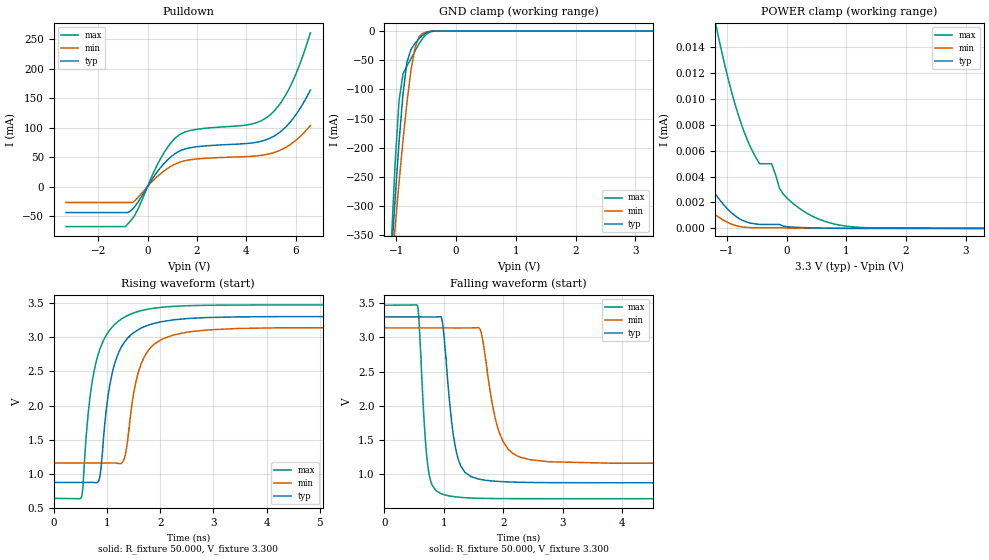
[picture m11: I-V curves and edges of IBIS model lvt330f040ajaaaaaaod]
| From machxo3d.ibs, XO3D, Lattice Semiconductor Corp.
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|   Model lvt330f040ajaaaaaaod
[Model] lvt330f040ajaaaaaaod
Model_type I/O_open_drain
Polarity   Non-Inverting
Enable   Active-Low
Vinl =  0.800V
Vinh =  2.000V
Vmeas =  1.650V
Cref =  0.0F
Rref = 10.00k
Vref = 3.30V
C_comp   4.200pF   3.800pF   7.500pF
[Temperature Range]   25.000   0.105k   -40.000
[Voltage Range]   3.300V   3.140V   3.470V
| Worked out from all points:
|   slope of the pulldown table from 0 to 0.495 V, typ, clamps not added: 16.2 ohm
|   GND clamp passes 1 mA (typ) near -0.43 V on its own axis
|   rising waveform, R_fixture 50.000, V_fixture 3.300: 20-80 % time 324ps typ, 329ps min, 328ps max; typ from 0.878 V to 3.3 V
|   falling waveform, R_fixture 50.000, V_fixture 3.300: 20-80 % time 180ps typ, 267ps min, 117ps max; typ from 3.3 V to 0.878 V
[Pulldown]
|Voltage   I(typ)   I(min)   I(max)
-3.3V     -43.98mA   -26.85mA   -67.81mA
-900mV    -43.98mA   -26.85mA   -67.81mA
-500mV    -33.06mA   -23.42mA   -47.39mA
600mV     35.86mA    24.47mA    52.84mA
1.2V      58.2mA     39.81mA    85.22mA
1.9V      67.18mA    46.53mA    96.69mA
4.2V      73.98mA    51.49mA    106.1mA
4.9V      81.14mA    55.32mA    119.6mA
5.4V      93.79mA    62.3mA     142.5mA
5.8V      110.5mA    71.89mA    171.7mA
6.2V      134mA      85.76mA    211.4mA
6.6V      164mA      103.9mA    261.1mA
[GND_clamp]
|Voltage   I(typ)   I(min)   I(max)
-3.3V     -4.507A    -3.482A    -6.263A
-1.089V   -398.4mA   -420.6mA   -374.7mA
-1.022V   -290.7mA   -338.6mA   -230.6mA
-955mV    -191.3mA   -260.2mA   -120mA
-888mV    -107.5mA   -187mA     -73.64mA
-821mV    -52.96mA   -121.4mA   -59.79mA
-754mV    -31.36mA   -66.92mA   -47.4mA
-687mV    -21.12mA   -28.79mA   -34.18mA
-620mV    -13.16mA   -10.19mA   -21.93mA
-553mV    -6.814mA   -3.53mA    -11.64mA
-352mV    -96.36uA   -46.21uA   -149.8uA
3.3V      0A         0A         0A
[POWER_clamp]
|Voltage   I(typ)   I(min)   I(max)
-3.3V     732.2uA    455.9uA    1.265mA
-2.663V   69.44uA    15.46uA    306.8uA
-2.529V   27.69uA    10.95uA    164.1uA
-2.328V   15.69uA    8.497uA    64.68uA
-1.725V   7.348uA    3.693uA    30.69uA
-1.189V   2.632uA    1.04uA     15.85uA
-988mV    1.494uA    463nA      11.72uA
-519mV    342.8nA    54.74nA    5.51uA
-251mV    305.1nA    47.61nA    4.994uA
-50mV     169nA      47.61nA    2.616uA
352mV     50.67nA    4.149nA    1.135uA
3.3V      0A         0A         0A
[Ramp]
| variable   typ   min   max
dV/dt_r   1.453/0.326n   1.187/0.327n   1.694/0.328n
dV/dt_f   1.453/0.179n   1.187/0.264n   1.694/0.117n
R_load = 50.000
[Rising Waveform]
R_fixture= 50.000
V_fixture= 3.300
V_fixture_min= 3.140
V_fixture_max= 3.470
|time   V(typ)   V(min)   V(max)
0s        878.1mV    1.161V     645.8mV
527ps     878.1mV    1.161V     681.6mV
672ps     878.8mV    1.161V     2.071V
842ps     898.9mV    1.161V     2.769V
1.041ns   2.249V     1.162V     3.094V
1.292ns   2.883V     1.171V     3.274V
1.542ns   3.088V     2.344V     3.364V
1.759ns   3.17V      2.786V     3.406V
3.465ns   3.295V     3.126V     3.468V
20ns      3.3V       3.14V      3.47V
[Falling Waveform]
R_fixture= 50.000
V_fixture= 3.300
V_fixture_min= 3.140
V_fixture_max= 3.470
|time   V(typ)   V(min)   V(max)
0s        3.3V       3.14V      3.47V
558ps     3.3V       3.14V      3.465V
745ps     3.298V     3.14V      1.041V
971ps     3.251V     3.14V      713.4mV
1.109ns   1.949V     3.14V      683.1mV
1.355ns   1.031V     3.14V      660.5mV
1.612ns   928.5mV    3.115V     651.6mV
1.999ns   893.9mV    1.477V     647.6mV
2.443ns   882.9mV    1.216V     646.1mV
20ns      878mV      1.161V     645.7mV
